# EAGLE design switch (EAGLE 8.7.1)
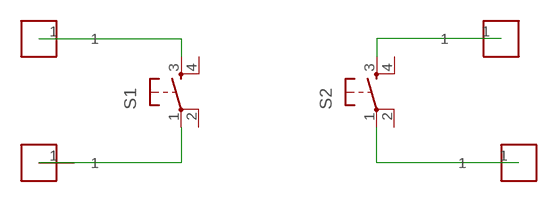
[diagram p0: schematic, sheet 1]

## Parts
PAD1  SOLDER_PAD  [SOLDERI_PAD]
PAD2  SOLDER_PAD  [SOLDERI_PAD]
PAD3  SOLDER_PAD  [SOLDERI_PAD]
PAD4  SOLDER_PAD  [SOLDERI_PAD]
S1  6MM_SWITCH6MM_SWITCH  [6MM_SWITCH]
S2  6MM_SWITCH6MM_SWITCH  [6MM_SWITCH]

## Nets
N$1: PAD1.1 S1.3(S)
N$2: PAD2.1 S1.1(P)
N$3: PAD3.1 S2.3(S)
N$4: PAD4.1 S2.1(P)
Unconnected: S1.2(P1) S1.4(S1) S2.2(P1) S2.4(S1)

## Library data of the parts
PAD1-PAD4 = doyo:SOLDER_PAD
S1 S2 = fab:6MM_SWITCH: OMRON SWITCH

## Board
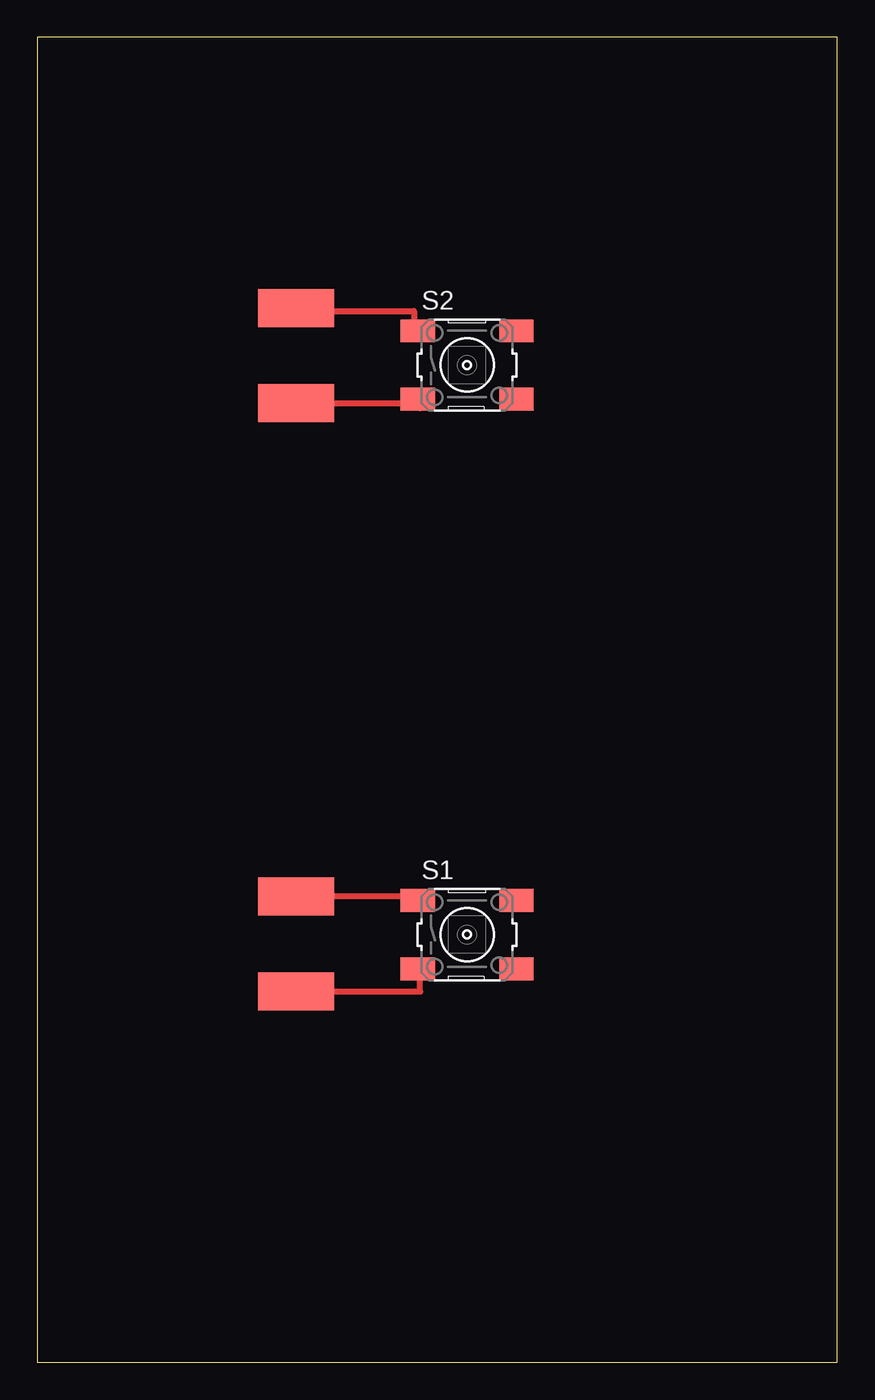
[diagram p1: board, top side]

Size 53.52 x 88.62 mm. Coordinates in mm from the lower left corner, seen from the top.
Outline: 0,0 53.52,0 53.52,88.62 0,88.62 0,0
Copper layers (1*16): Top 0.035mm / dielectric 1.5mm / Bottom 0.035mm
Design rules "default": minimum track width 6mil, minimum drill 0.35mm, track to track 6mil, track to pad 6mil, pad to pad 6mil, via to via 6mil, smd to smd 6mil, copper to edge 40mil, drill to drill 6mil, minimum pad ring 10mil, minimum via ring 8mil, stop-mask expansion 4mil, vias tented up to drill 0mil, thermal gap 10mil

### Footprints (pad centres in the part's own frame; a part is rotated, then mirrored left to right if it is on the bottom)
SOLDERI_PAD = smd 2.54 x 5.08: 1 0,0
6MM_SWITCH = smd 2.286 x 1.524: 1 -3.302,2.286; 2 3.302,2.286; 3 -3.302,-2.286; 4 3.302,-2.286

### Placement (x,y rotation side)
PAD1  17.32,24.79 90 top
PAD2  17.32,31.14 90 top
PAD3  17.32,64.16 90 top
PAD4  17.32,70.51 90 top
S1  28.75,28.6 0 top
S2  28.75,66.7 0 top

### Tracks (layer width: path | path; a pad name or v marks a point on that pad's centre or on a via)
N$1
  Top 0.406: PAD1.1 25.6,24.79 25.6,26.16 S1.3
N$2
  Top 0.406: PAD2.1 25.2,31.14 S1.1
N$3
  Top 0.406: PAD3.1 25.25,64.16 25.45,63.96 | 25.6,63.8 25.45,63.96 | 25.45,63.96 S2.3
N$4
  Top 0.406: PAD4.1 17.53,70.31 25.2,70.31 25.2,69.09 24.79,68.68 25.15,68.68 S2.1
